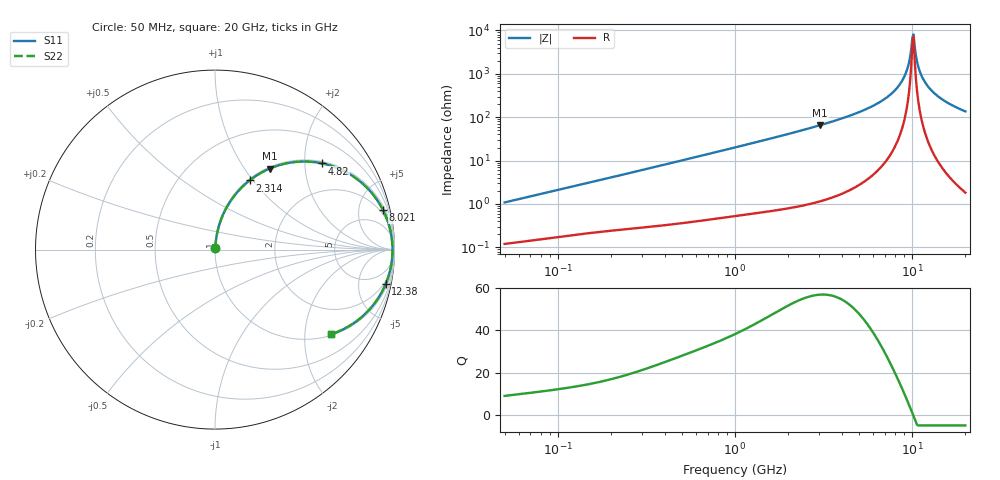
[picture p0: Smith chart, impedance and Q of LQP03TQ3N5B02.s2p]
!Murata Part Number: LQP03TQ3N5B02
!These Parameters are Measured in Series Mode Connection
!  o--[Z]--o
!Port1  Port2
!  o-------o
!Freq. Start=50[MHz] Stop=20[GHz], 401[Steps]
# Hz S RI R 50
!Freq.(Hz) S11(Real) S11(Imag) S21(Real) S21(Imag) S12(Real) S12(Imag) S22(Real) S22(Imag)
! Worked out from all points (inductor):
!   401 points, 50 MHz to 20 GHz, reference 50 ohm
!   read as one part in series: L = 3.4 nH near 51.52 MHz
!   highest Q = 56.9 at 3.03 GHz (marker M1), where L = 3.45 nH
!   self-resonance near 10.04 GHz
!   S11 on the Smith chart (normalised r, x): 50 MHz: 1.00, +0.02; 2.314 GHz: 1.02, +0.96; 4.82 GHz: 1.05, +2.45; 8.021 GHz: 1.43, +8.43; 12.38 GHz: 1.51, -9.87; 20 GHz: 1.04, -2.72
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5e7  0.00132 0.0108  0.9987 -0.0108  0.9987 -0.0108  0.00132 0.0108
1.364002e8  0.00282 0.0282  0.9972 -0.0282  0.9972 -0.0282  0.00282 0.0282
3.721004e8  0.0087 0.0743  0.9913 -0.0743  0.9913 -0.0743  0.0087 0.0743
1e9  0.0434 0.1911  0.9566 -0.1911  0.9566 -0.1911  0.0434 0.1911
2.313601e9  0.1929 0.3854  0.8071 -0.3854  0.8071 -0.3854  0.1929 0.3854
2.728004e9  0.2556 0.4274  0.7444 -0.4274  0.7444 -0.4274  0.2556 0.4274
3.029571e9  0.304 0.4513  0.696 -0.4513  0.696 -0.4513  0.304 0.4513
4.81993e9  0.5988 0.4801  0.4012 -0.4801  0.4012 -0.4801  0.5988 0.4801
6.125241e9  0.777 0.4033  0.223 -0.4033  0.223 -0.4033  0.777 0.4033
7.442007e9  0.9008 0.2799  0.0992 -0.2799  0.0992 -0.2799  0.9008 0.2799
8.020766e9  0.9369 0.2192  0.0631 -0.2192  0.0631 -0.2192  0.9369 0.2192
8.644534e9  0.9643 0.1527  0.0357 -0.1527  0.0357 -0.1527  0.9643 0.1527
9.178299e9  0.9792 0.0965  0.0208 -0.0965  0.0208 -0.0965  0.9792 0.0965
9.600142e9  0.986 0.0531  0.014 -0.0531  0.014 -0.0531  0.986 0.0531
9.892087e9  0.9884 0.0239  0.0116 -0.0239  0.0116 -0.0239  0.9884 0.0239
1.019291e10  0.989 -0.00547  0.011 0.00547  0.011 0.00547  0.989 -0.00547
1.034674e10  0.9887 -0.0201  0.0113 0.0201  0.0113 0.0201  0.9887 -0.0201
1.082228e10  0.9851 -0.064  0.0149 0.064  0.0149 0.064  0.9851 -0.064
1.115139e10  0.9805 -0.0929  0.0195 0.0929  0.0195 0.0929  0.9805 -0.0929
1.238412e10  0.9515 -0.1903  0.0485 0.1903  0.0485 0.1903  0.9515 -0.1903
1.504638e10  0.8521 -0.3427  0.1479 0.3427  0.1479 0.3427  0.8521 -0.3427
2e10  0.6474 -0.4711  0.3526 0.4711  0.3526 0.4711  0.6474 -0.4711
